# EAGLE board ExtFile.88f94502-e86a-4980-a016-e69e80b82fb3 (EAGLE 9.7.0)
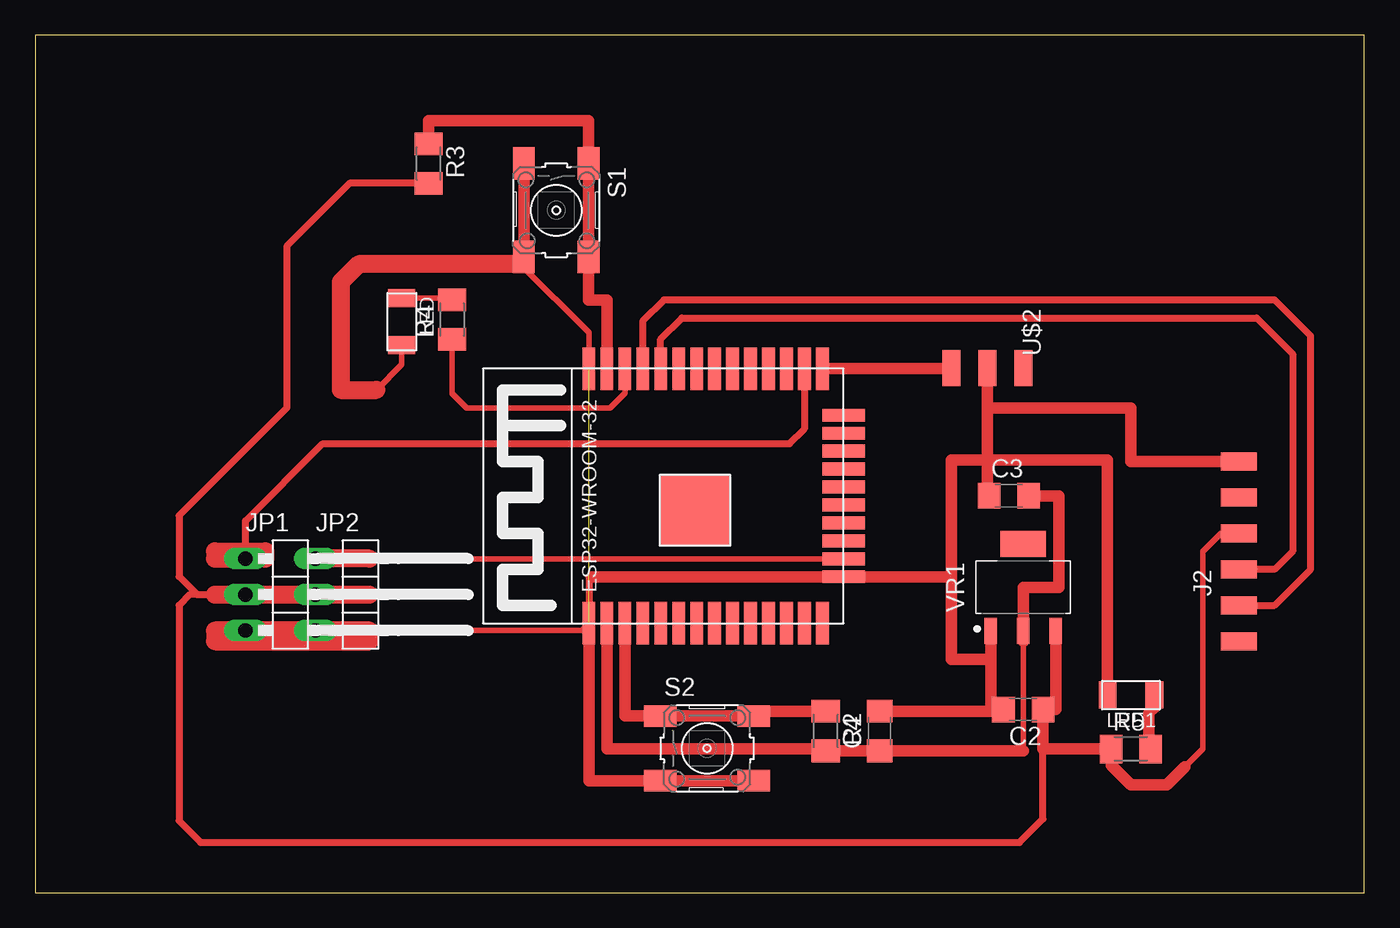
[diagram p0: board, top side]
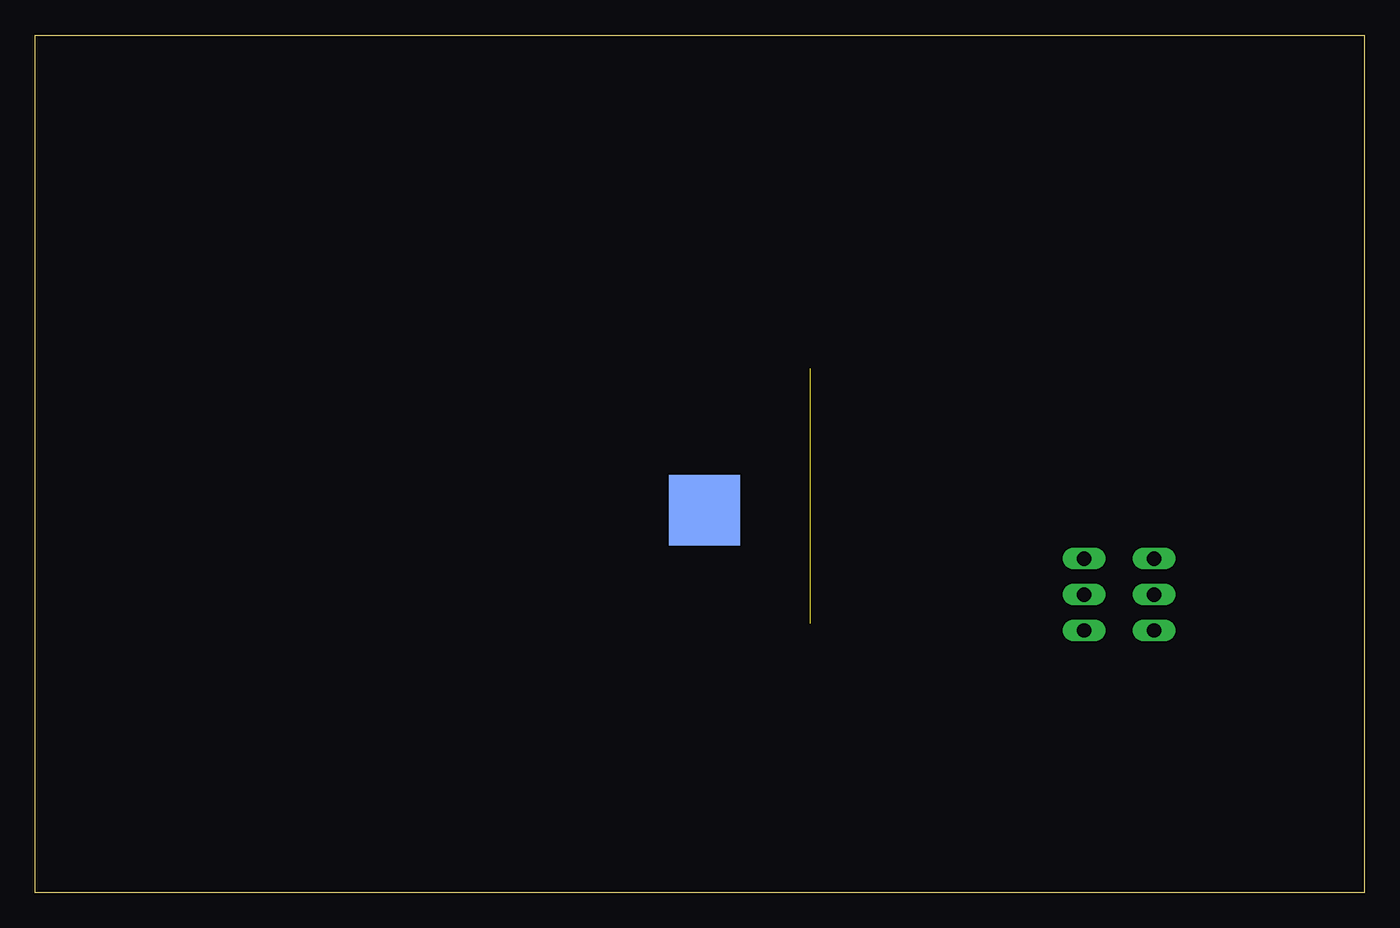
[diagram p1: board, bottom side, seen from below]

Size 93.96 x 60.63 mm. Coordinates in mm from the lower left corner, seen from the top.
Outline: 0,0 93.96,0 93.96,60.63 0,60.63 0,0
Copper layers (1*16): Top 0.05mm / dielectric 1.5mm / Bottom 0.05mm
Design rules "fabmodule *": minimum track width 10mil, minimum drill 0.4mm, track to track 0.42mm, track to pad 0.42mm, pad to pad 0.42mm, via to via 0.42mm, smd to smd 0.42mm, copper to edge 40mil, drill to drill 0.8mm, minimum pad ring 10mil, minimum via ring 8mil, stop-mask expansion 4mil, vias tented up to drill 0mil, thermal gap 10mil

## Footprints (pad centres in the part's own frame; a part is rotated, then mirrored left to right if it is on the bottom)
C1206 = smd 1.6 x 1.8: 1 -1.4,0; 2 1.4,0
1X06SMD = smd 2.54 x 1.27: 1 0,6.35; 2 0,3.81; 3 0,1.27; 4 0,-1.27; 5 0,-3.81; 6 0,-6.35
1X03/90 = drill 1.016 long: 1 -2.54,-3.81; 2 0,-3.81; 3 2.54,-3.81
LED1206FAB = smd 1.27 x 1.905: 1 -1.651,0; 2 1.651,0
M1206 = smd 1.6 x 2: 1 -1.4,0; 2 1.4,0
6MM_SWITCH = smd 2.286 x 1.524: 1 -3.302,2.286; 2 3.302,2.286; 3 -3.302,-2.286; 4 3.302,-2.286
ESP32-WROOM = smd 3 x 0.9: 3V3 0,16.74; EN 0,15.47; GND1 0,18.01; GND3 18,18.01; IO0 18,1.5; IO4 18,2.77; IO5 18,6.58; IO12 0,1.5; IO14 0,2.77; IO16 18,4.04; IO17 18,5.31; IO18 18,7.85; IO19 18,9.12; IO21 18,11.66; IO22 18,15.47; IO23 18,16.74; IO25 0,6.58; IO26 0,5.31; IO27 0,4.04; IO32 0,9.12; IO33 0,7.85; IO34 0,11.66; IO35 0,10.39; NC 18,10.39; RX 18,12.93; SENSOR_VN 0,12.93; SENSOR_VP 0,14.2; TX 18,14.2 | smd 0.9 x 3: CLK 9.635,0; CMD 8.365,0; GND2 3.285,0; IO2 14.715,0; IO13 4.555,0; IO15 13.445,0; SD0 10.905,0; SD1 12.175,0; SD2 5.825,0; SD3 7.095,0 | smd 5 x 5: GND4 8,10.5 | smd 5 x 5 bottom: GND5 8,10.5
SPDTSWITCH = smd 2.54 x 1.27: 1 0.38,2.54; 2 0.38,0; 3 0.38,-2.54
SOT230P700X170-4 = smd 1.86 x 0.898: 1 -3.075,2.3; 2 -3.075,0; 3 -3.075,-2.3 | smd 1.86 x 3.189: 4 3.075,0

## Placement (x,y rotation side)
C2  10uF  [C1206]  69.85,12.95 180 top
C3  1uF  [C1206]  68.83,28.07 0 top
C4  1uF  [C1206]  59.69,11.43 90 top
J2  FTDI-SMD-HEADER  [1X06SMD]  85.09,24.13 0 top
JP1  PINHD-1X3/90  [1X03/90]  18.67,21.08 270 top
JP2  PINHD-1X3/90  [1X03/90]  23.62,21.08 270 top
LED  LEDFAB1206  [LED1206FAB]  25.91,40.39 270 top
LED1  LEDFAB1206  [LED1206FAB]  77.47,13.97 180 top
R2  10k  [M1206]  55.88,11.43 270 top
R3  10k  [M1206]  27.81,51.56 270 top
R4  100  [M1206]  29.46,40.52 90 top
R5  100  [M1206]  77.47,10.16 0 top
S1  [6MM_SWITCH]  36.83,48.26 270 top
S2  [6MM_SWITCH]  47.5,10.2 0 top
U$1  ESP32-WROOM  [ESP32-WROOM]  57.15,19.05 90 top
U$2  SPDTSWITCH  [SPDTSWITCH]  67.31,37.46 270 top
VR1  NCP1117ST33T3G  [SOT230P700X170-4]  69.85,21.59 90 top

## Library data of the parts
C2-C4 R2-R5 = rcl
J2 LED LED1 S1 S2 U$2 = fab
JP1 JP2 = Connector; CATEGORY: CONNECTOR; SUB-CATEGORY: PIN-HEADER
U$1 = ESP32
VR1 = IC_Power-Management; CATEGORY: IC_Power-Management; MANUFACTURER: ON Semiconductor; MPN: NCP1117ST33T3G; OPERATING_TEMP: 0 to +125 °C; PART_STATUS: Active; ROHS_COMPLIANT: RoHS3 Compliant; SERIES: NCP1117, NCV1117; SUB-CATEGORY: Voltage Regulator; TYPE: Linear

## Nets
3.3V: C3.2 C4.1 R2.2 U$1.3V3 VR1.2
BUTTON: R3.1 S1.1 S1.2 U$1.IO23
CTS: J2.2
EN: R2.1 S2.1 S2.2 U$1.EN
GND: C2.2 C3.1 C4.2 J2.1 JP1.3 JP2.3 LED1.2 LED.2 S1.3 S1.4 S2.3 S2.4 U$1.GND1 U$1.GND2 U$1.GND3 U$2.2 VR1.1
LED_R: R4.1 U$1.IO22
N$1: LED1.1 R5.2
N$2: LED.1 R4.2
ONEWIRE: JP1.1 U$1.IO4
PROG_RUN: U$1.IO0 U$2.3
RTS: J2.6
RXD: J2.5 U$1.TX
SCL: U$1.IO15
SDA: U$1.IO14
SERVO: JP2.1 U$1.IO13
T5: U$1.IO12
TXD: J2.4 U$1.RX
VCC: C2.1 J2.3 JP1.2 JP2.2 R3.2 R5.1 VR1.3

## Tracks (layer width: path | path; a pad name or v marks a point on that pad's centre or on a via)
3.3V
  Top 0.406: 69.85,10.03 69.85,17.78 VR1.2 | 40.41,10.03 40.41,10.16
  Top 0.813: U$1.3V3 40.41,10.16 55.88,10.16 R2.2 C4.1 69.85,10.03 | C3.2 72.39,28.07 72.39,21.59 69.85,21.59 69.85,17.78
BUTTON
  Top 0.21: 27.86,53.16 R3.1 | 38.75,51.71 S1.1
  Top 0.813: U$1.IO23 40.41,41.91 39.12,41.91 S1.2 S1.1 39.12,54.61 27.81,54.61 27.81,53.16 27.86,53.16
EN
  Top 0.508: 41.91,12.49 41.68,12.49
  Top 0.813: 41.68,12.49 U$1.EN | 41.91,12.49 S2.1 S2.2 50.8,12.83 R2.1
GND  (1 unrouted)
  Top 0.406: U$1.GND3 39.14,39.6 34.29,44.45 34.29,44.7 S1.4 | 23.62,18.54 38.63,18.54 U$1.GND1 | 24.13,35.56 25.91,37.34 LED.2
  Top 0.508: U$1.GND1 39.14,22.34 39.37,22.34
  Top 0.813: U$1.GND1 39.14,7.92 S2.3 S2.4 | 64.77,22.34 U$1.GND2 39.37,22.34 | 64.77,22.34 64.77,30.61 67.31,30.61 | C3.1 67.31,28.07 67.31,30.61 | 67.31,30.61 67.31,34.29 | VR1.1 67.55,16.51 | 67.55,16.51 67.55,12.95 C2.2 68.45,12.83 C4.2 | 64.77,22.34 64.77,16.51 67.55,16.51 | 39.14,38.1 U$1.GND3 | S1.4 S1.3 | 67.31,34.29 77.47,34.29 77.47,30.48 J2.1 | 67.31,34.29 U$2.2 | 67.31,30.61 75.82,30.61 LED1.2
  Top 1.27: 24.13,35.56 21.59,35.56 21.59,43.18 22.86,44.45 34.04,44.45 S1.4 | 23.62,18.54 JP2.3 JP1.3 12.7,18.54 12.7,17.78 23.62,17.78 23.62,18.54
LED_R
  Top 0.406: R4.1 29.46,35.31 30.48,34.29 40.64,34.29 41.68,35.33 U$1.IO22
N$1
  Top 0.813: LED1.1 79.12,13.08 78.74,12.7 78.74,10.29 R5.2
N$2
  Top 0.406: LED.1 29.35,42.04 R4.2
  Top 0.813: R4.2 29.46,42.04
ONEWIRE
  Top 0.508: U$1.IO4 54.38,32.79 53.34,31.75 20.32,31.75 14.86,26.29 JP1.1
  Top 1.27: 12.7,23.62 JP1.1 16.26,23.62 16.26,24.13 12.7,24.13 12.7,23.62
PROG_RUN
  Top 0.813: U$1.IO0 64.77,37.05 U$2.3
RXD
  Top 0.508: J2.5 87.63,20.32 90.17,22.86 90.17,39.37 87.63,41.91 46.99,41.91 45.49,41.91 44.45,41.91 42.95,40.41 U$1.TX
SERVO
  Top 0.406: U$1.IO13 23.64,23.6 23.62,23.62
  Top 1.27: 23.62,23.62 JP2.1
TXD
  Top 0.508: J2.4 87.63,22.86 88.9,24.13 88.9,38.1 86.36,40.64 45.72,40.64 44.22,39.14 U$1.RX
VCC
  Top 0.406: 71.25,10.16 71.12,10.03 | 19.56,3.56 20.32,3.56 | J2.3 83.82,25.4 82.55,24.13 82.55,10.16 80.64,8.25
  Top 0.508: 11.43,21.08 12.7,21.08 | 11.43,21.08 10.92,21.08 10.16,20.32 10.16,5.08 11.68,3.56 20.32,3.56 69.6,3.56 71.25,5.21 71.25,10.16 | R3.2 22.22,50.16 17.78,45.72 17.78,34.29 10.16,26.67 10.16,22.35 11.43,21.08
  Top 0.813: VR1.3 72.15,12.95 C2.1 71.25,10.16 R5.1 76.07,9.02 77.47,7.62 80.01,7.62 80.64,8.25 81.28,8.89
  Top 1.27: 23.62,21.08 JP2.2 JP1.2 12.7,21.08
